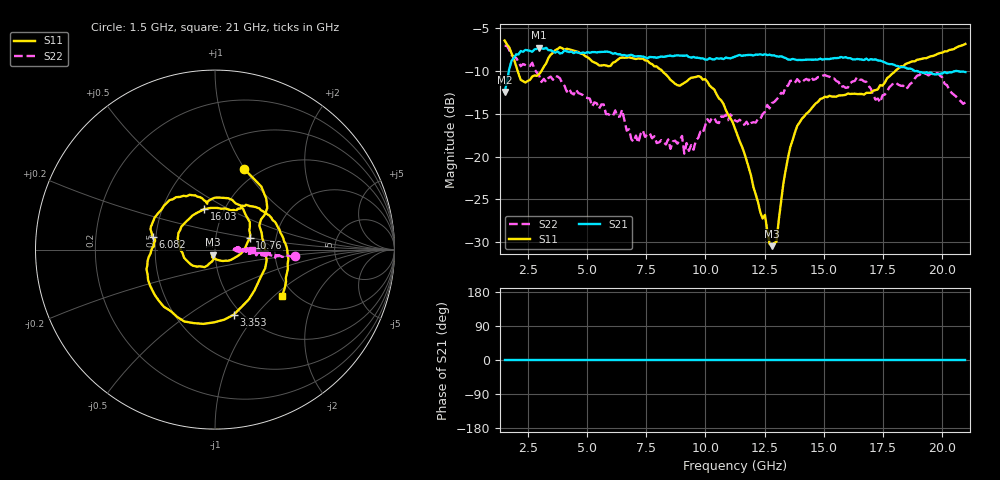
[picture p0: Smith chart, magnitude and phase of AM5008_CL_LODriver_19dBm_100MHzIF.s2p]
!Keysight Technologies,N5245B,MY58422270,A.16.20.02
!Mixer S2P File: Scalar Mixer Measurement
!Calibration State: On
!Parameters: Stimulus Freq, S11, SC21, SC12, S22
# Hz  S  DB  R  50.0
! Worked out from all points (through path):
!   201 points, 1.5 GHz to 21 GHz, reference 50 ohm
!   highest |S21| = -7.25 dB at 2.962 GHz (marker M1); lowest = -12.4 dB at 1.5 GHz (marker M2)
!   lowest |S11| = -30.5 dB at 12.81 GHz (marker M3), VSWR 1.06, Z = 48.9 - j2.75 ohm
!   |S11| at or under -10 dB: 2.054 GHz to 3.06 GHz (1.006 GHz wide, 39.3 % of centre); 8.173 GHz to 18.03 GHz (9.859 GHz wide, 75.2 % of centre)
!   |S22| runs from -19.6 to -7.0 dB; largest |S21 - S12| = 0.43
!   S11 on the Smith chart (normalised r, x): 1.5 GHz: 0.86, +1.00; 3.353 GHz: 0.92, -0.78; 6.082 GHz: 0.48, +0.08; 10.76 GHz: 1.46, +0.19; 16.03 GHz: 0.80, +0.38; 21 GHz: 1.74, -1.13
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1.5e9  -6.42 70.1  -12.45 0.0  -200.00 90.0  -7.04 -4.4
1.7925e9  -7.91 44.8  -8.82 0.0  -200.00 90.0  -8.16 -4.1
2.1825e9  -11.04 28.5  -7.65 0.0  -200.00 90.0  -9.43 -5.5
2.9625e9  -10.36 -38.0  -7.25 0.0  -200.00 90.0  -10.53 -5.0
3.3525e9  -8.47 -74.0  -7.56 0.0  -200.00 90.0  -10.80 -3.4
4.1325e9  -7.39 -131.7  -7.69 0.0  -200.00 90.0  -12.41 -1.3
4.815e9  -8.02 -164.0  -7.82 0.0  -200.00 90.0  -12.81 -6.8
6.0825e9  -9.02 168.8  -7.97 0.0  -200.00 90.0  -15.25 0.1
8.0325e9  -9.71 112.3  -8.37 0.0  -200.00 90.0  -18.34 -2.0
9.69e9  -10.59 75.5  -8.44 0.0  -200.00 90.0  -17.83 0.5
1.07625e10  -13.84 18.1  -8.60 0.0  -200.00 90.0  -15.34 -1.9
1.125e10  -16.71 -8.6  -8.32 0.0  -200.00 90.0  -15.78 -3.2
1.281e10  -30.47 -110.5  -8.17 0.0  -200.00 90.0  -13.74 -5.7
1.3005e10  -29.95 -103.4  -8.27 0.0  -200.00 90.0  -13.33 -0.4
1.359e10  -18.88 -120.9  -8.68 0.0  -200.00 90.0  -11.14 -6.0
1.4565e10  -14.10 175.3  -8.68 0.0  -200.00 90.0  -11.02 -5.5
1.60275e10  -12.62 104.9  -8.48 0.0  -200.00 90.0  -11.92 -3.4
1.64175e10  -12.69 92.6  -8.59 0.0  -200.00 90.0  -10.70 -5.0
1.73925e10  -11.65 60.7  -8.77 0.0  -200.00 90.0  -13.65 -4.1
1.77825e10  -10.63 55.8  -9.19 0.0  -200.00 90.0  -11.89 -4.0
1.983e10  -7.98 2.2  -10.36 0.0  -200.00 90.0  -10.24 -4.3
2.1e10  -6.82 -34.5  -10.11 0.0  -200.00 90.0  -13.67 -0.1
